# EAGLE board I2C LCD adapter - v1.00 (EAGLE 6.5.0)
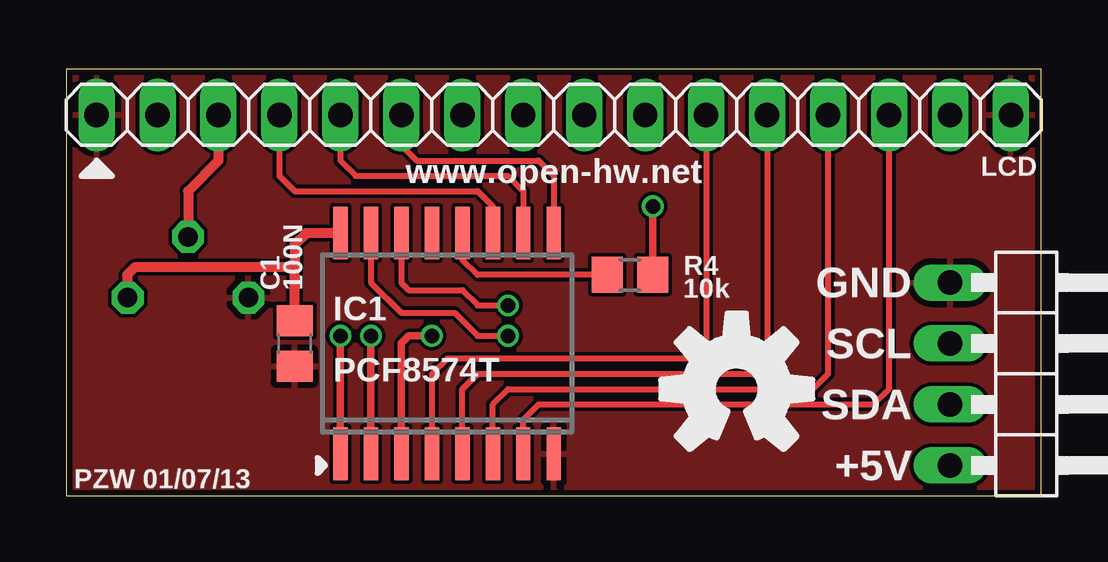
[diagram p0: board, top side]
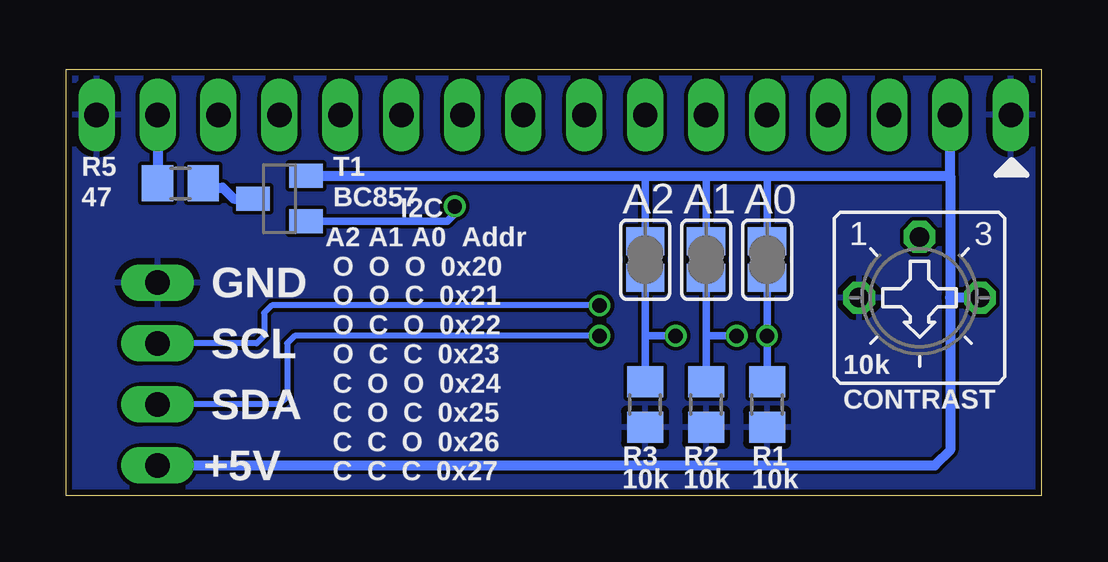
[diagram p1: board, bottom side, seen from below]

Size 40.64 x 17.78 mm. Coordinates in mm from the lower left corner, seen from the top.
Outline: 0,0 40.64,0 40.64,17.78 0,17.78 0,0
Copper layers (1*16): Top 0.035mm / dielectric 1.5mm / Bottom 0.035mm
Design rules "ITEADstudio_DRC": minimum track width 6mil, minimum drill 12mil, track to track 6mil, track to pad 6mil, pad to pad 6mil, via to via 6mil, smd to smd 0mil, copper to edge 10mil, drill to drill 10mil, minimum pad ring 10mil, minimum via ring 6mil, stop-mask expansion 2mil, vias tented up to drill 100mil, thermal gap 10mil

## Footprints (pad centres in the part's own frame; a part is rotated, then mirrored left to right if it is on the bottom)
SJ = smd 1.168 x 1.6: 1 -0.762,0; 2 0.762,0
C0805 = smd 1.3 x 1.5: 1 -0.95,0; 2 0.95,0
CT6 = drill 0.813 octagon: A 2.515,0; E -2.515,0; S 0,-2.54
SO16W = smd 0.6 x 2.2: 1 -4.445,-4.6; 2 -3.175,-4.6; 3 -1.905,-4.6; 4 -0.635,-4.6; 5 0.635,-4.6; 6 1.905,-4.6; 7 3.175,-4.6; 8 4.445,-4.6; 9 4.445,4.6; 10 3.175,4.6; 11 1.905,4.6; 12 0.635,4.6; 13 -0.635,4.6; 14 -1.905,4.6; 15 -3.175,4.6; 16 -4.445,4.6
1X04/90 = drill 1.016 long: 1 -3.81,-3.81; 2 -1.27,-3.81; 3 1.27,-3.81; 4 3.81,-3.81
1X16 = drill 1.016 long: 1 -19.05,0; 2 -16.51,0; 3 -13.97,0; 4 -11.43,0; 5 -8.89,0; 6 -6.35,0; 7 -3.81,0; 8 -1.27,0; 9 1.27,0; 10 3.81,0; 11 6.35,0; 12 8.89,0; 13 11.43,0; 14 13.97,0; 15 16.51,0; 16 19.05,0
R0805 = smd 1.3 x 1.5: 1 -0.95,0; 2 0.95,0
SOT23-BEC = smd 1 x 1.4: B -0.95,-1.1; C 0,1.1; E 0.95,-1.1

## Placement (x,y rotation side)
A0  [SJ]  11.43,9.84 270 bottom
A1  [SJ]  13.97,9.84 270 bottom
A2  [SJ]  16.51,9.84 270 bottom
C1  100N  [C0805]  9.53,6.35 270 top
CONTRAST  10k  [CT6]  5.08,8.26 180 bottom
IC1  PCF8574T  [SO16W]  15.88,6.35 0 top
JP1  [1X04/90]  40.64,5.08 270 top
LCD  [1X16]  20.32,15.88 0 top
R1  10k  [R0805]  11.43,3.81 90 bottom
R2  10k  [R0805]  13.97,3.81 90 bottom
R3  10k  [R0805]  16.51,3.81 90 bottom
R4  10k  [R0805]  23.5,9.21 0 top
R5  47  [R0805]  35.88,13.02 180 bottom
T1  BC857  [SOT23-BEC]  31.75,12.38 90 bottom

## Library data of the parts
A0 A1 A2 = jumper
C1 R1-R5 = rcl
CONTRAST = work
IC1 = micro-philips; MPN: PCF8574T/3,512; OC_FARNELL: 1201255; OC_NEWARK: 70R6870
JP1 LCD = pinhead
T1 = transistor-pnp

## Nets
GND: C1.2 CONTRAST.A IC1.8 JP1.1 LCD.1 LCD.16 R1.1 R2.1 R3.1
N$1: IC1.14 JP1.2
N$2: IC1.15 JP1.3
N$3: A0.2 IC1.1 R1.2
N$4: A1.2 IC1.2 R2.2
N$5: A2.2 IC1.3 R3.2
N$6: IC1.12 R4.1
N$7: R5.1 T1.C
N$8: R4.2 T1.B
N$9: LCD.15 R5.2
N$10: CONTRAST.S LCD.3
N$11: IC1.4 LCD.11
N$12: IC1.5 LCD.12
N$13: IC1.6 LCD.13
N$14: IC1.7 LCD.14
N$15: IC1.9 LCD.6
N$16: IC1.10 LCD.5
N$17: IC1.11 LCD.4
VCC: A0.1 A1.1 A2.1 C1.1 CONTRAST.E IC1.16 JP1.4 LCD.2 T1.E

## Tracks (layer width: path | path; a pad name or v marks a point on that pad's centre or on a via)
GND
  pour Bottom: 0,0 40.64,0 40.64,17.78 0,17.78
  pour Top: 0,0 40.64,0 40.64,17.78 0,17.78
N$1  (via drill 0.6)
  Top 0.254: IC1.14 13.97,8.89 14.29,8.57 16.51,8.57 17.14,7.94 v18.41,7.94
  Bottom 0.254: v18.41,7.94 32.07,7.94 32.38,7.62 32.38,6.67 32.7,6.35 JP1.2
N$2  (via drill 0.6)
  Top 0.254: IC1.15 12.7,8.89 13.97,7.62 16.19,7.62 17.14,6.67 v18.41,6.67
  Bottom 0.254: v18.41,6.67 31.11,6.67 31.43,6.35 31.43,4.13 31.75,3.81 JP1.3
N$3  (via drill 0.6)
  Top 0.305: IC1.1 v11.43,6.67
  Bottom 0.305: R1.2 v11.43,6.67 A0.2
N$4  (via drill 0.6)
  Top 0.305: IC1.2 v12.7,6.67
  Bottom 0.305: A1.2 13.97,6.67 | 13.97,6.67 R2.2 | v12.7,6.67 13.97,6.67
N$5  (via drill 0.6)
  Top 0.305: IC1.3 13.97,6.35 14.29,6.67 v15.24,6.67
  Bottom 0.305: A2.2 16.51,6.67 | 16.51,6.67 R3.2 | v15.24,6.67 16.51,6.67
N$6
  Top 0.254: R4.1 17.14,9.21 16.51,9.84 IC1.12
N$7
  Bottom 0.406: T1.C 33.66,12.38 34.12,12.85 34.76,12.85 R5.1
N$8  (via drill 0.6)
  Top 0.305: v24.45,12.06 24.45,9.53 R4.2
  Bottom 0.305: T1.B 24.76,11.43 24.45,11.75 v24.45,12.06
N$9
  Bottom 0.406: LCD.15 R5.2
N$10
  Top 0.406: LCD.3 6.35,13.97 5.08,12.7 CONTRAST.S
N$11
  Top 0.254: LCD.11 26.67,6.35 26.04,5.71 15.88,5.71 15.24,5.08 IC1.4
N$12
  Top 0.254: IC1.5 16.51,4.45 17.14,5.08 28.57,5.08 29.21,5.71 LCD.12
N$13
  Top 0.254: IC1.6 17.78,3.81 18.41,4.45 31.11,4.45 31.75,5.08 LCD.13
N$14
  Top 0.254: IC1.7 19.05,3.17 19.68,3.81 33.66,3.81 34.29,4.45 LCD.14
N$15
  Top 0.254: LCD.6 13.97,14.61 14.61,13.97 19.68,13.97 20.32,13.34 IC1.9
N$16
  Top 0.254: LCD.5 11.43,13.97 12.06,13.34 18.41,13.34 19.05,12.7 IC1.10
N$17
  Top 0.254: LCD.4 8.89,13.34 9.53,12.7 17.14,12.7 17.78,12.06 IC1.11
VCC
  Top 0.406: C1.1 9.53,9.53 | 9.53,9.53 2.86,9.53 2.54,9.21 2.54,8.28 CONTRAST.E | IC1.16 10,10.95 9.53,10.48 9.53,9.53
  Bottom 0.305: A0.1 11.43,13.34 | A2.1 16.51,13.34 | A1.1 13.97,13.34
  Bottom 0.406: JP1.4 4.45,1.27 3.81,1.91 3.81,8.26 | 3.81,13.34 LCD.2 | 3.81,13.34 11.43,13.34 13.97,13.34 16.51,13.34 T1.E | 3.81,13.34 3.81,8.26 | CONTRAST.E 3.81,8.26

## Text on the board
tNames: www.open-hw.net | GND | SCL | SDA | +5V | PZW 01/07/13
bNames: GND | SCL | SDA | I2C / A2 A1 A0 Addr / O O O 0x20 / O O C 0x21 / O C O 0x22 / O C C 0x23 / C O O 0x24 / C O C 0x25 / C C O 0x26 / C C C 0x27 | +5V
